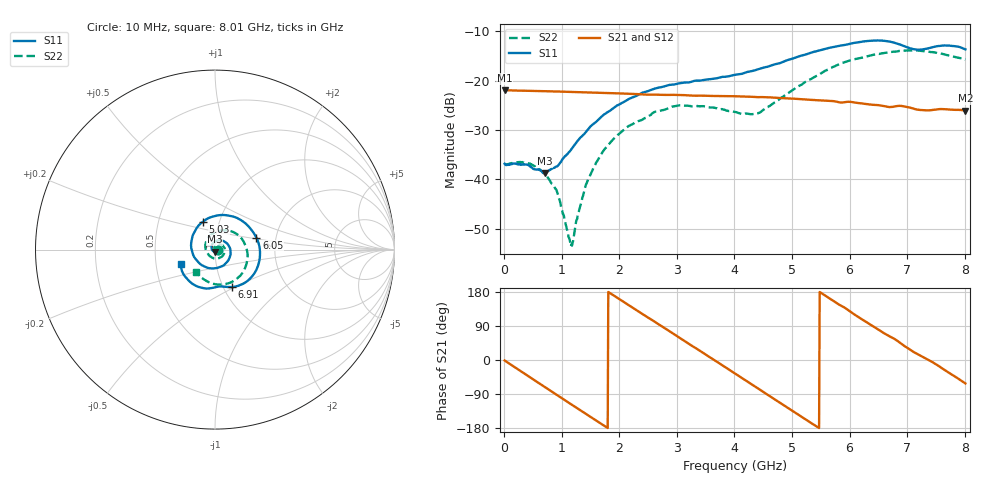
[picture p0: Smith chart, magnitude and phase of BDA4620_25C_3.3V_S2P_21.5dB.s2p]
!Agilent Technologies,E5071B,MY42404982,A.09.10
!Date: Wed May 06 08:53:24 2026
!Data & Calibration Information:
!Freq	S11:SOLT2(ON)	S21:SOLT2(ON)	S12:SOLT2(ON)	S22:SOLT2(ON)
# Hz S RI R 50
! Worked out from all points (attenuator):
!   801 points, 10 MHz to 8.01 GHz, reference 50 ohm
!   highest |S21| = -21.90 dB at 10 MHz (marker M1); lowest = -26.1 dB at 8.01 GHz (marker M2)
!   lowest |S11| = -38.8 dB at 710 MHz (marker M3), VSWR 1.02, Z = 49.7 - j1.12 ohm
!   |S11| at or under -10 dB: start of sweep to end of sweep
!   |S22| runs from -53.5 to -13.8 dB; largest |S21 - S12| = 0.00041
!   S11 on the Smith chart (normalised r, x): 10 MHz: 1.03, -0.00; 5.03 GHz: 0.83, +0.27; 6.05 GHz: 1.58, +0.23; 6.91 GHz: 1.10, -0.48; 8.01 GHz: 0.67, -0.12
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1e7  0.0144 -0.000947  0.0803 -0.00171  0.0804 -0.00169  0.0141 -0.000499
4.4e8  0.00841 -0.0109  0.0564 -0.0554  0.0565 -0.0556  0.0135 -0.00524
7.1e8  -0.00265 -0.0112  0.0249 -0.0744  0.0248 -0.0746  0.00855 -0.00731
9.3e8  -0.0123 -0.00583  -0.00462 -0.0777  -0.00477 -0.0778  0.00332 -0.0064
1.16e9  -0.0188 0.00652  -0.0342 -0.0691  -0.0344 -0.0692  -0.00174 -0.00118
1.2e9  -0.0193 0.00918  -0.0388 -0.0665  -0.0389 -0.0665  -0.00238 -4.08e-06
1.35e9  -0.0191 0.0196  -0.0543 -0.054  -0.0544 -0.054  -0.00397 0.00468
1.53e9  -0.0136 0.0329  -0.0676 -0.0346  -0.0677 -0.0346  -0.00378 0.0115
1.77e9  0.00239 0.0468  -0.0751 -0.00445  -0.0752 -0.00452  0.000538 0.021
2.15e9  0.0413 0.0497  -0.0613 0.0414  -0.0614 0.0415  0.0173 0.0298
2.68e9  0.0851 0.00254  -0.00574 0.072  -0.00571 0.0721  0.0451 0.0196
3.07e9  0.0768 -0.0561  0.0396 0.0598  0.0398 0.0598  0.056 -0.00682
4.01e9  -0.0817 -0.0807  0.0565 -0.0407  0.0566 -0.0409  -0.0111 -0.0471
4.42e9  -0.1315 0.00425  0.0164 -0.0663  0.0164 -0.0665  -0.0455 -0.0129
5.03e9  -0.0678 0.1551  -0.0478 -0.0453  -0.0479 -0.0454  -0.0286 0.0767
5.35e9  0.0281 0.1922  -0.0626 -0.0133  -0.0627 -0.0133  0.0231 0.1033
6.05e9  0.2307 0.0673  -0.0335 0.0506  -0.0336 0.0507  0.1548 0.0524
6.37e9  0.2469 -0.063  -0.00254 0.0574  -0.00249 0.0574  0.1803 -0.0162
6.68e9  0.1768 -0.1779  0.0241 0.0486  0.0241 0.0487  0.171 -0.0917
6.91e9  0.0938 -0.2087  0.0416 0.0367  0.0417 0.0367  0.1429 -0.1426
7.57e9  -0.0814 -0.211  0.0491 -0.0163  0.0491 -0.0162  -0.0178 -0.1884
8.01e9  -0.1916 -0.0822  0.0235 -0.0438  0.0235 -0.0439  -0.1037 -0.1268
